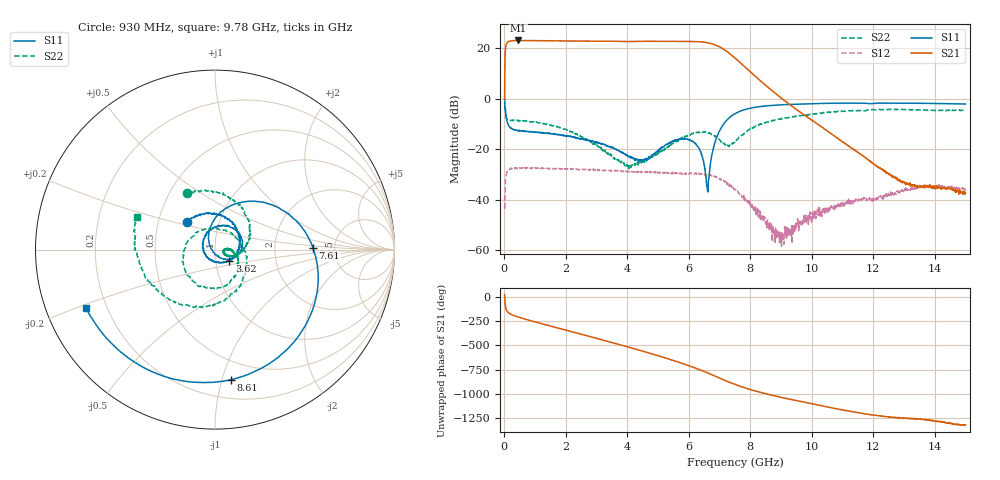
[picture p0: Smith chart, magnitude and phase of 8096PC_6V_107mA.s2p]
!Keysight Technologies,N5247B,US58420632,A.15.75.19
!Date: Wednesday, November 02, 2022 15:39:30
!Correction: S11(C  2-Port  )
!S21(C  2-Port  )
!S12(C  2-Port  )
!S22(C  2-Port  )
!S2P File: Measurements: S11, S21, S12, S22:
# Hz S  dB  R 50
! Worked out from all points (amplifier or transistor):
!   1500 points, 10 MHz to 15 GHz, reference 50 ohm
!   highest |S21| = 23.1 dB at 460 MHz (marker M1)
!   |S21| within 3 dB of that: 40.26 MHz to 7.072 GHz (7.031 GHz wide, 198 % of centre)
!   unconditionally stable (mu >= 1): 11.52 MHz to end of sweep
!   at 2.51 GHz: K = 1.14, MAG = 23.2 dB, |S12| = -28.0 dB
!   at 7.51 GHz: K = 3.68, MAG = 17.5 dB, |S12| = -36.0 dB
!   at 15 GHz: K = 568.82, MAG = -31.3 dB, |S12| = -35.9 dB
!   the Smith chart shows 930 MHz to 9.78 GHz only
!   S11 on the Smith chart (normalised r, x): 930 MHz: 0.70, +0.23; 3.62 GHz: 1.16, -0.15; 7.61 GHz: 3.40, +0.09; 8.61 GHz: 0.34, -1.07; 9.78 GHz: 0.12, -0.21
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1e7  -1.64 -33.0  -0.21 22.6  -43.58 154.2  0.06 -37.4
9e7  -8.95 -111.9  22.20 -148.1  -29.07 51.8  -8.28 -145.2
1.6e8  -10.95 -139.8  22.78 -170.5  -28.03 23.9  -8.61 -165.1
4.6e8  -12.77 172.5  23.10 149.7  -27.29 -22.5  -8.78 156.3
9.3e8  -13.17 135.1  23.05 106.9  -27.51 -60.2  -9.14 116.3
1.83e9  -14.36 78.1  22.94 30.3  -27.69 -130.2  -11.54 51.8
2.51e9  -15.94 39.2  22.84 -26.8  -27.97 178.7  -15.11 6.7
3.09e9  -17.51 1.8  22.83 -76.2  -28.09 134.6  -19.07 -17.5
3.62e9  -19.92 -37.7  22.77 -122.4  -28.41 90.7  -23.78 -28.1
4.34e9  -24.28 -119.3  22.71 174.4  -28.88 33.6  -25.27 -5.0
5.01e9  -20.27 124.1  22.74 111.6  -29.38 -23.4  -21.39 1.9
5.52e9  -16.55 64.7  22.73 61.2  -29.27 -67.7  -17.75 -18.9
6.1e9  -16.80 -0.8  22.68 -0.8  -29.67 -124.6  -13.87 -66.7
6.74e9  -22.94 121.9  21.82 -81.3  -30.40 165.8  -14.05 -149.9
7.12e9  -10.32 60.1  19.75 -134.2  -32.60 121.4  -17.64 129.5
7.51e9  -5.85 11.8  16.11 176.2  -35.98 79.2  -17.11 21.8
7.61e9  -5.26 1.0  15.01 164.6  -37.36 71.5  -15.63 -2.2
8.61e9  -2.73 -83.1  4.22 72.9  -48.74 20.6  -9.04 -119.7
9.78e9  -2.06 -155.7  -6.62 -8.2  -48.72 69.8  -6.54 157.6
1.001e10  -1.98 -168.6  -8.49 -23.4  -45.50 55.2  -6.01 142.7
1.251e10  -1.71 61.6  -30.04 -158.9  -37.95 -78.8  -4.22 -1.8
1.5e10  -2.07 -65.8  -37.35 120.8  -35.93 133.6  -4.56 -141.0
